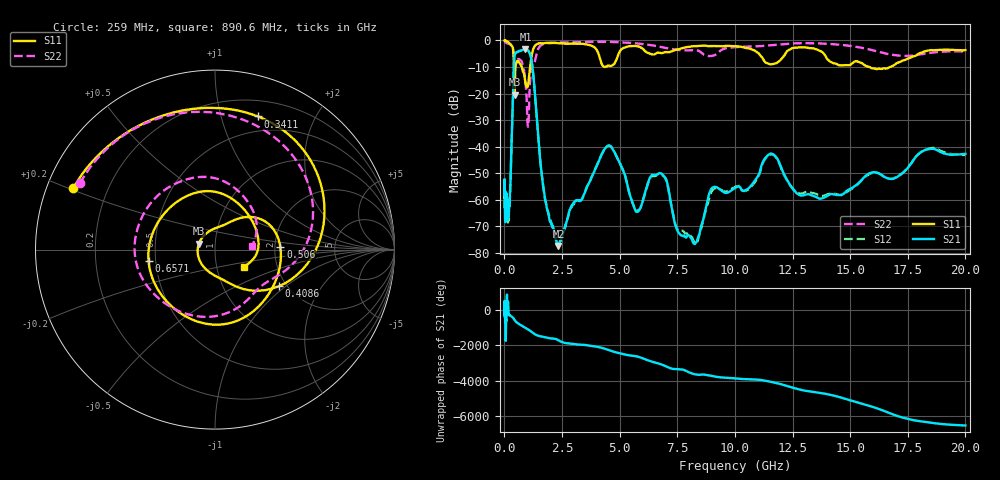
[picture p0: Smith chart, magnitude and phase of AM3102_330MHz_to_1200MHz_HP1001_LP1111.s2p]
! Date/Time: Tue, Sep 11, 2018 5:18 PM
! Network Analyzer: Agilent Technologies E8362B Rev: A.07.50.63
! Sweep from 0.010 to 20.000 GHz, 1601 Points, Sweep Type: LOG
! Power Supply: 4.949 V, 0.001 A
# Hz S DB R 50
!freq MagS11 AngS11 MagS21 AngS21 MagS12 AngS12 MagS22 AngS22
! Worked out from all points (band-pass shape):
!   1601 points, 10 MHz to 20 GHz, reference 50 ohm
!   highest |S21| = -3.22 dB at 916.3 MHz (marker M1); lowest = -77.5 dB at 2.347 GHz (marker M2)
!   |S21| within 3 dB of the highest: 436.8 MHz to 1.146 GHz (708.9 MHz wide, 89.6 % of centre)
!   lowest |S11| = -20.4 dB at 443 MHz (marker M3), VSWR 1.21, Z = 41.7 + j2.74 ohm
!   |S11| at or under -10 dB: 415.3 MHz to 481.7 MHz (66.4 MHz wide, 14.8 % of centre); 758.1 MHz to 1.116 GHz (357.8 MHz wide, 38.2 % of centre); 15.84 GHz to 16.73 GHz (891.5 MHz wide, 5.47 % of centre)
!   |S22| runs from -32.5 to -0.2 dB; largest |S21 - S12| = 0.0092
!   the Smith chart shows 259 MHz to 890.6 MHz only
!   S11 on the Smith chart (normalised r, x): 259 MHz: 0.08, +0.21; 341.1 MHz: 0.35, +1.31; 408.6 MHz: 1.81, -0.89; 506 MHz: 2.14, +0.06; 657.1 MHz: 0.46, -0.07; 890.6 MHz: 1.35, -0.27
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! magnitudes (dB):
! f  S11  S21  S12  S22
! 10 MHz  0.0  -53.2  -53.0  -0.2
! 35.55 MHz  0.0  -62.9  -65.4  -0.5
! 126.4 MHz  -0.4  -64.2  -64.6  -1.1
! 259 MHz  -1.3  -54.7  -54.7  -1.5
! 341.1 MHz  -2.2  -30.0  -30.1  -2.4
! 408.6 MHz  -7.8  -10.4  -10.4  -6.0
! 443 MHz  -20.4  -5.8  -5.8  -9.6
! 447.2 MHz  -20.1  -5.5  -5.6  -9.7
! 506 MHz  -8.8  -4.5  -4.6  -8.3
! 657.1 MHz  -8.5  -3.9  -4.0  -7.1
! 890.6 MHz  -14.6  -3.3  -3.3  -13.7
! 916.3 MHz  -16.0  -3.2  -3.3  -15.8
! 1.027 GHz  -16.8  -3.8  -3.8  -32.5
! 1.59 GHz  -1.1  -48.1  -48.1  -1.8
! 2.347 GHz  -1.0  -77.5  -77.0  -0.8
! 4.479 GHz  -9.6  -39.8  -39.7  -0.5
! 5.652 GHz  -2.1  -63.4  -63.1  -1.0
! 6.771 GHz  -4.7  -50.0  -50.4  -2.4
! 8.149 GHz  -2.2  -75.2  -74.2  -3.7
! 11.53 GHz  -9.0  -42.7  -43.0  -1.8
! 13.94 GHz  -6.0  -58.9  -58.2  -1.2
! 20 GHz  -3.6  -42.7  -43.2  -4.2
